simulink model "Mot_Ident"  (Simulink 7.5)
settings: Solver=ode3  StartTime=0.0  StopTime=inf  FixedStep=Ts  RelTol=1e-3
PreLoadFcn:
  | Ts=0.01;
  | comPorts=arduino.Prefs.searchForComPort
  | arduino.Prefs.setComPort(comPorts{1});
libraries: simulink x6, arduino_lib x5

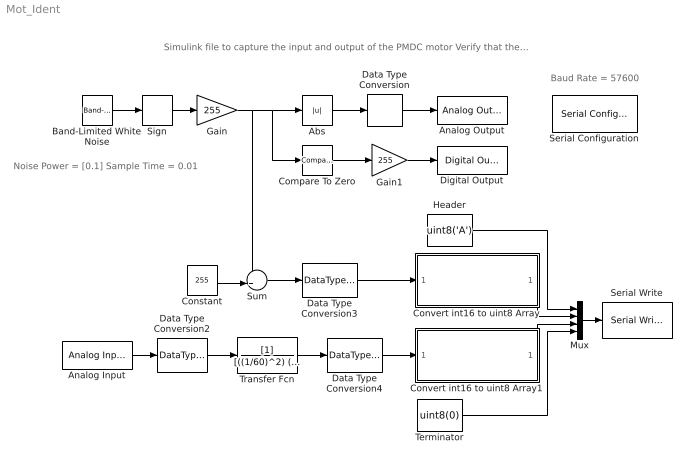
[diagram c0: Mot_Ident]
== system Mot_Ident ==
  note: Noise Power = [0.1] Sample Time = 0.01
  note: Baud Rate = 57600
  note: Simulink file to capture the input and output of the PMDC motor Verify that the sampling time 'Ts = 0.01' is set in the workspace
  Abs : Abs  OutDataType=fixdt(1, 16)  OutScaling=2^0
  Analog Input : arduino_lib/Analog Input  SParameter1=0  SampleTime=Ts
  Analog Output : arduino_lib/Analog Output  SParameter1=6  SampleTime=-1
  Band-Limited White Noise : simulink/Sources/Band-Limited White Noise  SystemSampleTime=-1  Cov=[0.1]  Ts=Ts  seed=[23341]
  Compare To Zero : simulink/Logic and Bit Operations/Compare To Zero  SystemSampleTime=-1  relop=<=  LogicOutDataTypeMode=boolean
  Constant : Constant  Value=255  OutDataType=fixdt(1, 16)  OutScaling=2^0
  Convert int16 to uint8 Array : Subsystem
  Convert int16 to uint8 Array1 : Subsystem
  Data Type Conversion : DataTypeConversion  OutDataTypeMode=uint8  OutDataType=fixdt(1, 16)  OutScaling=2^0  OutDataTypeStr=uint8
  Data Type Conversion2 : DataTypeConversion  OutDataTypeMode=double  OutDataType=fixdt(1, 16)  OutScaling=2^0  OutDataTypeStr=double
  Data Type Conversion3 : DataTypeConversion  OutDataTypeMode=int16  OutDataType=fixdt(1, 16)  OutScaling=2^0  OutDataTypeStr=int16
  Data Type Conversion4 : DataTypeConversion  OutDataTypeMode=int16  OutDataType=fixdt(1, 16)  OutScaling=2^0  OutDataTypeStr=int16
  Digital Output : arduino_lib/Digital Output  SParameter1=13  SampleTime=-1
  Gain : Gain  Gain=255  ParameterDataType=fixdt(1, 16)  ParameterScaling=2^0  OutDataType=fixdt(1, 16)  OutScaling=2^0
  Gain1 : Gain  Gain=255  ParameterDataType=fixdt(1, 16)  ParameterScaling=2^0  OutDataType=fixdt(1, 16)  OutScaling=2^0
  Header : Constant  Value=uint8('A')  OutDataType=fixdt(1, 16)  OutScaling=2^0
  Mux : Mux
  Serial Configuration : arduino_lib/Serial Configuration  SParameter1=57600
  Serial Write : arduino_lib/Serial Write  SampleTime=-1
  Sign : Signum
  Sum : Sum  Inputs=++|  OutDataType=fixdt(1, 16)  OutScaling=2^0
  Terminator : Constant  Value=uint8(0)  OutDataType=fixdt(1, 16)  OutScaling=2^0
  Transfer Fcn : TransferFcn  Denominator=[((1/60)^2) (2*0.707*(1/60)) 1]
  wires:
  Data Type Conversion/1 -> Analog Output/1
  Abs/1 -> Data Type Conversion/1
  Constant/1 -> Sum/2
  Sum/1 -> Data Type Conversion3/1
  Data Type Conversion3/1 -> Convert int16 to uint8 Array/1(From Analog In)
  Gain/1 -> Sum/1, Abs/1, Compare To Zero/1
  Transfer Fcn/1 -> Data Type Conversion4/1
  Data Type Conversion2/1 -> Transfer Fcn/1
  Analog Input/1 -> Data Type Conversion2/1
  Header/1 -> Mux/1
  Convert int16 to uint8 Array/1(To Serial) -> Mux/2
  Mux/1 -> Serial Write/1
  Convert int16 to uint8 Array1/1(To Serial) -> Mux/3
  Terminator/1 -> Mux/4
  Data Type Conversion4/1 -> Convert int16 to uint8 Array1/1(From Analog In)
  Sign/1 -> Gain/1
  Band-Limited White Noise/1 -> Sign/1
  Compare To Zero/1 -> Gain1/1
  Gain1/1 -> Digital Output/1

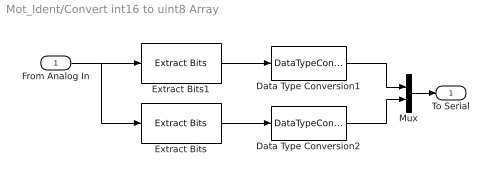
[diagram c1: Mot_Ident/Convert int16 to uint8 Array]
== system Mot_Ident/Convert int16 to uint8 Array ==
  From Analog In : Inport
  Data Type Conversion1 : DataTypeConversion  OutDataTypeMode=uint8  OutDataType=fixdt(1, 16)  OutScaling=2^0  OutDataTypeStr=uint8  ConvertRealWorld=Stored Integer (SI)
  Data Type Conversion2 : DataTypeConversion  OutDataTypeMode=uint8  OutDataType=fixdt(1, 16)  OutScaling=2^0  OutDataTypeStr=uint8  ConvertRealWorld=Stored Integer (SI)
  Extract Bits : simulink/Logic and Bit Operations/Extract Bits  SystemSampleTime=-1  bitsToExtract=Upper half  numBits=8  bitIdxRange=[0 7]  outScalingMode=Treat bit field as an integer
  Extract Bits1 : simulink/Logic and Bit Operations/Extract Bits  SystemSampleTime=-1  bitsToExtract=Lower half  numBits=8  bitIdxRange=[0 7]  outScalingMode=Treat bit field as an integer
  Mux : Mux  Inputs=2
  To Serial : Outport
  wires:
  Mux/1 -> To Serial/1
  Data Type Conversion2/1 -> Mux/2
  Data Type Conversion1/1 -> Mux/1
  Extract Bits/1 -> Data Type Conversion2/1
  Extract Bits1/1 -> Data Type Conversion1/1
  From Analog In/1 -> Extract Bits1/1, Extract Bits/1

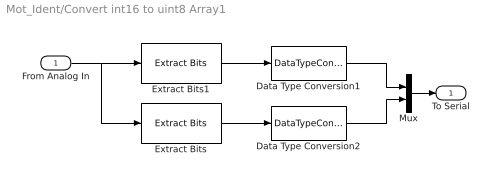
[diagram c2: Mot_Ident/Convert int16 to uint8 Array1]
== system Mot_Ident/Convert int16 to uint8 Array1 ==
  From Analog In : Inport
  Data Type Conversion1 : DataTypeConversion  OutDataTypeMode=uint8  OutDataType=fixdt(1, 16)  OutScaling=2^0  OutDataTypeStr=uint8  ConvertRealWorld=Stored Integer (SI)
  Data Type Conversion2 : DataTypeConversion  OutDataTypeMode=uint8  OutDataType=fixdt(1, 16)  OutScaling=2^0  OutDataTypeStr=uint8  ConvertRealWorld=Stored Integer (SI)
  Extract Bits : simulink/Logic and Bit Operations/Extract Bits  SystemSampleTime=-1  bitsToExtract=Upper half  numBits=8  bitIdxRange=[0 7]  outScalingMode=Treat bit field as an integer
  Extract Bits1 : simulink/Logic and Bit Operations/Extract Bits  SystemSampleTime=-1  bitsToExtract=Lower half  numBits=8  bitIdxRange=[0 7]  outScalingMode=Treat bit field as an integer
  Mux : Mux  Inputs=2
  To Serial : Outport
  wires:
  From Analog In/1 -> Extract Bits/1, Extract Bits1/1
  Extract Bits1/1 -> Data Type Conversion1/1
  Extract Bits/1 -> Data Type Conversion2/1
  Data Type Conversion1/1 -> Mux/1
  Data Type Conversion2/1 -> Mux/2
  Mux/1 -> To Serial/1
